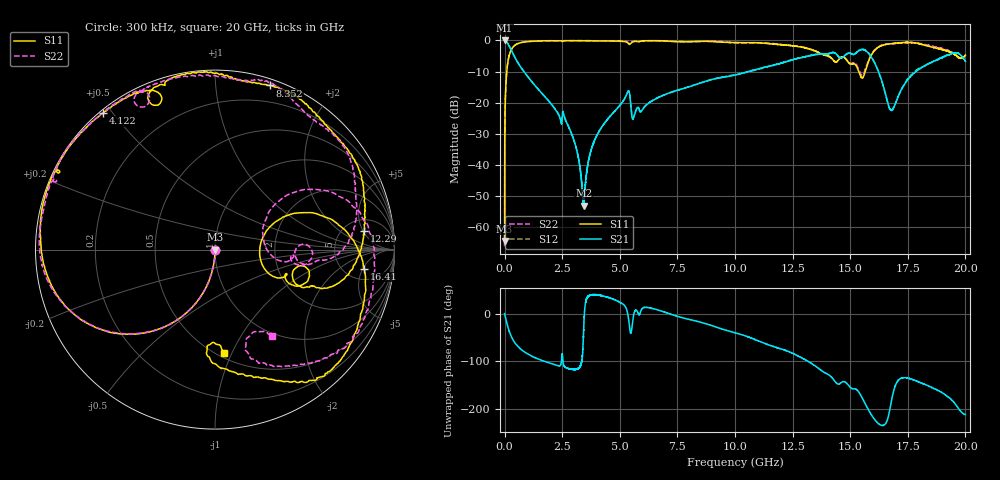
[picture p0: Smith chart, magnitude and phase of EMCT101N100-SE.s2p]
!EMCT101N100
!Johanson Technology Inc.
!www.johansontechnology.com
!Test Board Conditions:
!Substrate Type  RO4350B
!Substrate Thickness  10 mil
!Substrate Dk  3.66
!TL Type: GCPW
!TL Trace Width  22 mil
!TL Gap  14 mil
!PART MODE SINGLE ENDED (AKA BYPASS)
!DUT TOPOLOGY	SERIES-SHUNT
# MHz S  dB  R 50
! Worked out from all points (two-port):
!   20001 points, 300 kHz to 20 GHz, reference 50 ohm
!   highest |S21| = 0.00 dB at 1.3 MHz (marker M1); lowest = -53.1 dB at 3.432 GHz (marker M2)
!   |S21| within 3 dB of the highest: start of sweep to 282.1 MHz; 15.45 GHz to 15.6 GHz (156.4 MHz wide, 1.01 % of centre)
!   lowest |S11| = -64.6 dB at 300 kHz (marker M3), VSWR 1.00, Z = 50.1 - j0.00166 ohm
!   |S11| at or under -10 dB: start of sweep to 93.38 MHz; 15.37 GHz to 15.65 GHz (278.9 MHz wide, 1.8 % of centre)
!   |S22| runs from -66.2 to 0.0 dB; largest |S21 - S12| = 0.018
!   S11 on the Smith chart (normalised r, x): 300 kHz: 1.00, -0.00; 4.122 GHz: 0.01, +0.47; 8.352 GHz: 0.05, +1.39; 12.29 GHz: 7.70, +5.31; 16.41 GHz: 7.52, -5.30; 20 GHz: 0.54, -0.94
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0.3  -64.56 -1.6  -0.01 -0.1  0.01 -0.1  -66.22 46.0
1.3  -47.28 -86.6  0.00 -0.3  -0.00 -0.3  -47.14 -85.5
111.298  -8.66 -113.2  -0.67 -22.8  -0.67 -22.8  -8.69 -113.0
330.295  -2.48 -142.5  -3.74 -52.0  -3.71 -52.1  -2.52 -142.6
938.286  -0.43 -173.3  -11.01 -82.9  -11.06 -82.9  -0.32 -173.6
2608.261  -0.06 152.1  -24.92 -112.1  -24.89 -112.3  -0.09 155.6
3334.25  -0.08 139.7  -44.90 -104.6  -44.89 -102.9  -0.01 145.4
3432.249  -0.10 138.4  -53.15 -35.4  -52.95 -31.8  -0.03 144.4
4122.238  -0.14 129.3  -28.95 38.6  -28.93 38.6  -0.11 136.3
5333.22  -0.68 109.7  -16.71 2.2  -16.71 2.8  -0.49 113.3
5596.216  -0.38 111.5  -24.90 -3.8  -24.83 -3.3  -0.27 117.1
6667.2  -0.08 93.5  -18.38 7.4  -18.36 7.0  -0.15 105.3
8352.175  -0.31 71.4  -14.07 -16.2  -14.02 -16.7  -0.35 78.8
10000.15  -0.68 44.8  -11.13 -40.4  -10.98 -40.5  -0.74 57.3
12285.12  -1.53 7.0  -6.70 -79.1  -6.59 -79.4  -1.50 20.8
13334.1  -3.00 -15.6  -4.75 -105.3  -4.79 -105.5  -2.91 0.1
15540.07  -11.99 3.4  -2.89 -178.9  -2.80 -179.0  -11.09 15.7
16411.05  -1.54 -7.2  -13.90 124.9  -14.16 124.2  -1.42 11.1
16667.05  -1.16 -18.1  -20.98 145.9  -21.22 146.9  -1.08 1.2
18273.03  -1.59 -62.0  -8.01 -149.6  -7.98 -150.9  -1.40 -45.1
19495.01  -4.27 -92.4  -3.98 174.1  -4.12 174.5  -4.12 -71.9
20000  -4.71 -84.7  -6.74 147.8  -6.76 149.4  -4.68 -56.3
